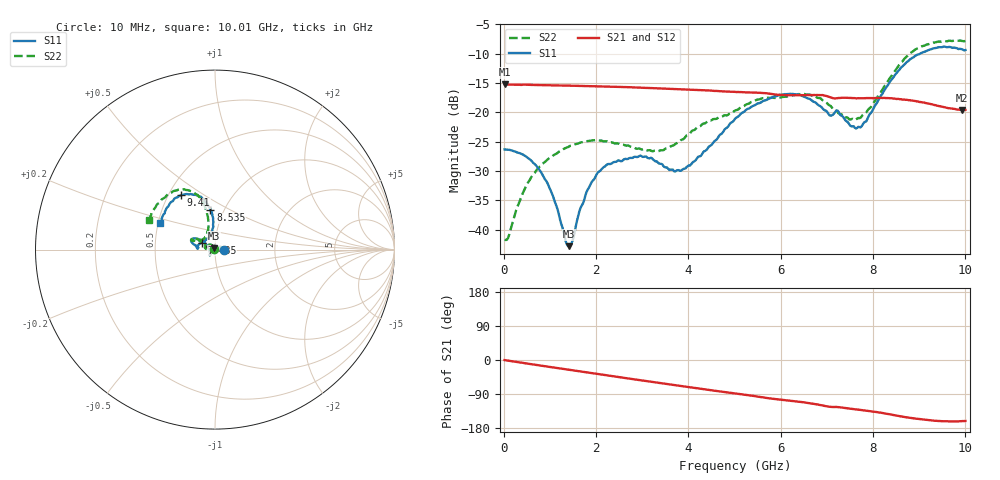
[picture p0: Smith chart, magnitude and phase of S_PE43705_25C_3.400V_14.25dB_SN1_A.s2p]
! Device ID: PE43705
! Serial: 1
! Insertion: A
! Impedance: 50 ohm
! Temp: 25C
! VDD: 3.400V
! Attenuation Step: 14.25dB
#  Hz  S  RI  R  50
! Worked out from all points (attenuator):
!   401 points, 10 MHz to 10.01 GHz, reference 50 ohm
!   highest |S21| = -15.24 dB at 10 MHz (marker M1); lowest = -19.6 dB at 9.935 GHz (marker M2)
!   lowest |S11| = -42.8 dB at 1.41 GHz (marker M3), VSWR 1.01, Z = 49.6 + j0.609 ohm
!   |S11| at or under -10 dB: start of sweep to 9.026 GHz
!   |S22| runs from -41.7 to -7.8 dB; largest |S21 - S12| = 0.0013
!   S11 on the Smith chart (normalised r, x): 10 MHz: 1.10, +0.00; 7.435 GHz: 0.86, +0.07; 8.535 GHz: 0.86, +0.40; 9.41 GHz: 0.58, +0.40; 10.01 GHz: 0.51, +0.17
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1e7  0.0484 0.000145  0.1729 -0.000707  0.173 -0.000676  -0.0082 0.000587
4.35e8  0.0415 0.0118  0.1704 -0.0246  0.1698 -0.0242  -0.0111 0.0187
7.6e8  0.0282 0.0163  0.1657 -0.0415  0.1656 -0.0415  -0.0211 0.0269
1.01e9  0.0159 0.0147  0.1611 -0.0545  0.1611 -0.0544  -0.03 0.0284
1.41e9  -0.00388 0.00614  0.152 -0.0734  0.1522 -0.0733  -0.0444 0.0257
1.685e9  -0.0158 -0.00312  0.1443 -0.0857  0.1444 -0.0856  -0.0517 0.0206
1.885e9  -0.0229 -0.0097  0.1381 -0.0941  0.1382 -0.094  -0.0552 0.0166
2.21e9  -0.0278 -0.0218  0.127 -0.1068  0.127 -0.1068  -0.0559 0.00988
2.935e9  -0.0292 -0.0309  0.0979 -0.1298  0.0981 -0.1298  -0.0484 0.00911
3.36e9  -0.0265 -0.0255  0.079 -0.1391  0.0792 -0.1387  -0.0453 0.0121
3.885e9  -0.0327 -0.00347  0.055 -0.1467  0.0553 -0.1466  -0.0536 0.0247
5.01e9  -0.0721 0.0507  0.00453 -0.1494  0.00469 -0.1494  -0.0887 0.0534
5.985e9  -0.1274 0.0602  -0.0348 -0.1364  -0.0342 -0.1364  -0.1191 0.0608
6.685e9  -0.1215 0.0316  -0.0596 -0.127  -0.0597 -0.1272  -0.1286 0.0512
7.435e9  -0.0738 0.0395  -0.0806 -0.106  -0.0803 -0.1061  -0.071 0.0563
7.76e9  -0.0343 0.0681  -0.0883 -0.0978  -0.0881 -0.098  -0.049 0.0788
8.36e9  -0.011 0.1787  -0.1061 -0.0789  -0.1054 -0.0793  -0.0416 0.1891
8.535e9  -0.0255 0.2195  -0.1095 -0.0705  -0.1087 -0.0711  -0.0552 0.2343
8.935e9  -0.0787 0.2945  -0.1128 -0.0532  -0.1125 -0.0523  -0.1238 0.3222
9.41e9  -0.1891 0.3032  -0.1076 -0.0372  -0.1074 -0.0373  -0.2318 0.3261
9.935e9  -0.2961 0.1755  -0.0991 -0.0336  -0.0997 -0.0333  -0.3556 0.1937
1.001e10  -0.3049 0.1483  -0.0992 -0.0344  -0.0991 -0.0347  -0.3704 0.1653
